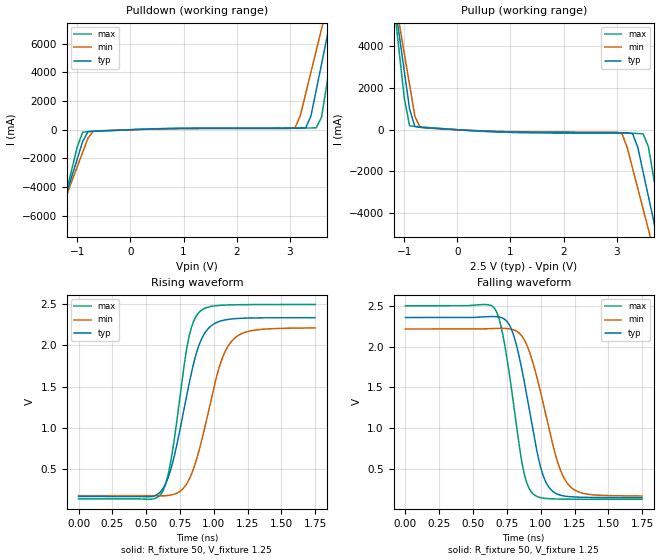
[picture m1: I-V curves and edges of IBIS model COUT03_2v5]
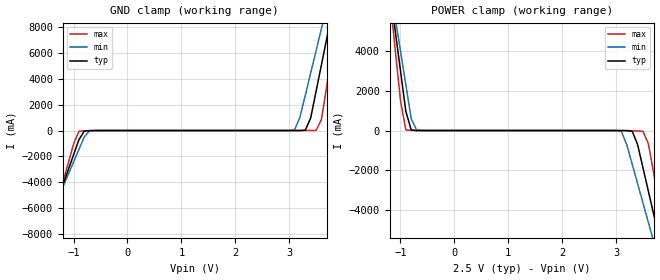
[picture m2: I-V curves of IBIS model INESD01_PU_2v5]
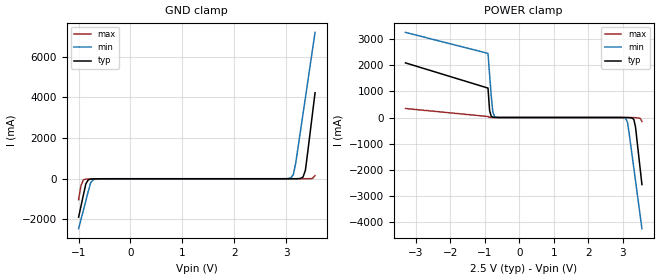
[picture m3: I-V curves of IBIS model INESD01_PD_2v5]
|   This file is an IBIS representation of the   |
|   Integrated Device Technology , Inc.   |
|   ICS8701   |
|   LOW SKEW div1, div2 CLOCK GENERATOR   |
[IBIS Ver]   4.1
[File name]   8701.ibs
[File Rev]   1.0
[Date]   24 Nov 2009 | Last modified
|   Aug 16 2000 | Generated
[Source]   Originated at Integrated Device Technology, Inc.
[Disclaimer]
IDT hereby grants the user of this IBIS model a non-exclusive,
nontransferable license to use this IBIS model under the following terms.
Before using this IBIS model, the user should read this license.
If the user does not accept these terms,  the IBIS model should be
returned to IDT within 30 days.
   The user is granted this license only to use the IBIS model and
is not granted rights to sell, load, rent, lease or license the IBIS
model in whole or in part, or in modified form to anyone other than
user. User may modify the IBIS model to suit its specific
applications but rights to derivative works and such modifications
shall belong to IDT.
   This IBIS model is provided on an "AS IS" basis and IDT makes
absolutely no warranty with respect to the information contained
herein. IDT DISCLAIMS AND CUSTOMER WAIVES ALL WARRANTIES, EXPRESS
OR IMPLIED, INCLUDING WARRANTIES OF MERCHANTABILITY OR FITNESS FOR
A PARTICULAR PURPOSE. The entire risk as to quality and performance
is with the Customer. ACCORDINGLY, IN NO EVENT SHALL THE COMPANY BE
LIABLE FOR ANY DAMAGES, WHETHER IN CONTRACT OR TORT,INCLUDING ANY
LOST PROFITS OR OTHER INCIDENTAL, CONSEQUENTIAL, EXEMPLARY, OR
PUNITIVE DAMAGES ARISING OUT OF THE USE OR APPLICATION OF THE IBIS
model provided in this package. Further, IDT reserves the right to
make changes without notice to any product herein to improve
reliability, function, or design. IDT does not convey any license
under patent rights or any other intellectual property rights,
including those of third parties.
   IDT is not obligated to provide maintenance or support
for the licensed IBIS model.
[Copyright]   Copyright 2002 by Integrated Device Technology , Inc.
[Component]   ICS8701Y
[Manufacturer] Integrated Device Technology, Inc.
[Package]
|LQFP48
|lead + wire   typ   min   max
R_pkg   220.4m   212.5m   238m
L_pkg   1.841nH   1.708nH   1.974n
C_pkg   0.316pF   0.2907pF   0.338pF
[Pin] signal_name   model_name   R_pin   L_pin   C_pin
1   QC3   COUT03   238m   1.974n   0.338p
2   VDDO   POWER   225m   1.831n   0.330p
3   QC4   COUT03   220m   1.781n   0.323p
4   QD0   COUT03   214m   1.732n   0.312p
5   VDDO   POWER   214m   1.709n   0.305p
6   QD1   COUT03   213m   1.708n   0.291p
7   GND   GND   213m   1.708n   0.291p
8   QD2   COUT03   214m   1.709n   0.305p
9   GND   GND   214m   1.732n   0.312p
10   QD3   COUT03   220m   1.781n   0.323p
11   VDDO   POWER   225m   1.831n   0.330p
12   QD4   COUT03   238m   1.974n   0.338p
13   DIV_SELD   INESD01_PU   238m   1.974n   0.338p
14   DIV_SELC   INESD01_PU   225m   1.831n   0.330p
15   nMR/OE   INESD01_PU   220m   1.781n   0.323p
16   VDD   POWER   214m   1.732n   0.312p
17   BANK_EN1   INESD01_PU   214m   1.709n   0.305p
18   GND   GND   213m   1.708n   0.291p
19   BANK_EN0   INESD01_PU   213m   1.708n   0.291p
20   VDD   POWER   214m   1.709n   0.305p
21   GND   GND   214m   1.732n   0.312p
22   CLK   INESD01_PD   220m   1.781n   0.323p
23   DIV_SELB   INESD01_PU   225m   1.831n   0.330p
24   DIV_SELA   INESD01_PU   238m   1.974n   0.338p
25   QA0   COUT03   238m   1.974n   0.338p
26   VDDO   POWER   225m   1.831n   0.330p
27   QA1   COUT03   220m   1.781n   0.323p
28   GND   GND   214m   1.732n   0.312p
29   QA2   COUT03   214m   1.709n   0.305p
30   GND   GND   213m   1.708n   0.291p
31   QA3   COUT03   213m   1.708n   0.291p
32   VDDO   POWER   214m   1.709n   0.305p
33   QA4   COUT03   214m   1.732n   0.312p
34   QB0   COUT03   220m   1.781n   0.323p
35   VDDO   POWER   225m   1.831n   0.330p
36   QB1   COUT03   238m   1.974n   0.338p
37   GND   GND   238m   1.974n   0.338p
38   QB2   COUT03   225m   1.831n   0.330p
39   GND   GND   220m   1.781n   0.323p
40   QB3   COUT03   214m   1.732n   0.312p
41   VDDO   POWER   214m   1.709n   0.305p
42   QB4   COUT03   213m   1.708n   0.291p
43   QC0   COUT03   213m   1.708n   0.291p
44   VDDO   POWER   214m   1.709n   0.305p
45   QC1   COUT03   214m   1.732n   0.312p
46   GND   GND   220m   1.781n   0.323p
47   QC2   COUT03   225m   1.831n   0.330p
48   GND   GND   238m   1.974n   0.338p
[Model Selector] COUT03
COUT03_2v5  Buffer selection for 2v5
COUT03_3v3  Buffer selection for 3v3
[Model Selector] INESD01_PU
INESD01_PU_2v5  Buffer selection for 2v5
INESD01_PU_3v3  Buffer selection for 3v3
[Model Selector] INESD01_PD
INESD01_PD_2v5  Buffer selection for 2v5
INESD01_PD_3v3  Buffer selection for 3v3
| Models and submodels in the file (6): COUT03_2v5 (Output), INESD01_PU_2v5 (Input), INESD01_PD_2v5 (Input), COUT03_3v3 (Output), INESD01_PU_3v3 (Input), INESD01_PD_3v3 (Input)
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[Model] COUT03_2v5
Model_type   Output
Polarity   Non-Inverting
|   typ   min   max
C_comp   2pF   1.5pF   2.5pF
Vmeas = 1.25V
Rref = 50
Cref = 0
Vref = 1.25V
|   typ   min   max
[Voltage range]   2.5V   2.375V   2.625V
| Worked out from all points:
|   slope of the pulldown table from 0 to 0.375 V, typ, clamps not added: 7.86 ohm
|   slope of the pullup table from 0 to 0.375 V, typ, clamps not added: 7.18 ohm
|   rising waveform, R_fixture 50, V_fixture 1.25: 20-80 % time 171ps typ, 188ps min, 123ps max; typ from 0.163 V to 2.34 V
|   falling waveform, R_fixture 50, V_fixture 1.25: 20-80 % time 153ps typ, 185ps min, 125ps max; typ from 2.35 V to 0.154 V
[Pulldown]
|Voltage   I (typ)   I (min)   I (max)
-3.3V     -29.21A    -25.24A    -35.89A
-1.5V     -7.924A    -7.485A    -8.724A
-1.4V     -6.739A    -6.498A    -7.212A
-900mV    -814mA     -1.56A     -170mA
-700mV    -98.53mA   -106.3mA   -114.1mA
3.1V      103.9mA    137.5mA    121.4mA
3.3V      129mA      2.499A     122mA
3.4V      958.9mA    4.006A     122.9mA
3.6V      4.58A      7.024A     878.2mA
3.7V      6.391A     8.534A     3.192A
3.9V      10.02A     11.55A     7.823A
6.6V      59.32A     52.62A     70.8A
[Pullup]
|Voltage   I (typ)   I (min)   I (max)
-3.3V     44.66A     38.54A     54.95A
-1.2V     6.458A     6.703A     6.17A
-1.1V     4.638A     5.186A     3.844A
-1V       2.817A     3.67A      1.518A
-900mV    996.3mA    2.153A     194.9mA
-700mV    116.1mA    120.7mA    136.7mA
3.1V      -144.3mA   -177.7mA   -168.5mA
3.4V      -851mA     -2.819A    -180.7mA
3.6V      -3.21A     -4.786A    -822.6mA
3.7V      -4.391A    -5.77A     -2.33A
3.9V      -6.753A    -7.739A    -5.346A
6.6V      -38.66A    -34.34A    -46.07A
[Ramp]
|   typ   min   max
dV/dt_r   1.743/0.263n   1.634/0.293n   1.896/0.19n
dV/dt_f   1.77/0.231n   1.639/0.28n   1.903/0.187n
R_load =   50.0000
[Rising Waveform]
R_fixture = 50
V_fixture = 1.25   |Vcc_typ
V_fixture_min = 1.1875 |Vcc_min
V_fixture_max = 1.3125 |Vcc_max
C_fixture = 0.0p
| Time   typ   min   max
0s        162.8mV    173.3mV    133.8mV
614.9ps   238.4mV    170.2mV    204.6mV
684.9ps   510.9mV    180.8mV    621.8mV
814.6ps   1.513V     361.6mV    2.092V
853.1ps   1.799V     516.4mV    2.304V
903.9ps   2.06V      804.5mV    2.423V
1.042ns   2.293V     1.748V     2.487V
1.142ns   2.324V     2.07V      2.494V
1.303ns   2.335V     2.187V     2.497V
1.748ns   2.337V     2.213V     2.498V
[Falling Waveform]
R_fixture = 50
V_fixture = 1.25   |Vcc_typ
V_fixture_min = 1.1875 |Vcc_min
V_fixture_max = 1.3125 |Vcc_max
C_fixture = 0.0p
| Time   typ   min   max
0s        2.355V     2.214V     2.498V
662.2ps   2.366V     2.222V     2.456V
721.7ps   2.345V     2.223V     2.13V
798.8ps   2.141V     2.205V     1.303V
874.1ps   1.606V     2.095V     474.6mV
949.5ps   917.4mV    1.762V     192.4mV
1.046ns   319.7mV    1.11V      143.2mV
1.128ns   193.6mV    572.7mV    137.3mV
1.203ns   167.9mV    316.2mV    135.5mV
1.748ns   154.2mV    174.5mV    133.9mV
[Model] INESD01_PU_2v5
Model_type   Input
Polarity   Non-Inverting
Vinl = 1.4V
Vinh = 1.85V
|   typ   min   max
C_comp   2pF   1.5pF   2.5pF
|   typ   min   max
[Voltage range]  2.5V   2.375V   2.625V
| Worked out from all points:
|   GND clamp passes 1 mA (typ) near -0.54 V on its own axis
|   POWER clamp passes 1 mA (typ) near -0.66 V on its own axis
[GND_clamp]
|Voltage   I(typ)   I(min)   I(max)
-2.5V     -19.6A     -17.18A    -23.67A
-1.6V     -8.969A    -8.332A    -10.1A
-1.5V     -7.788A    -7.349A    -8.588A
-900mV    -707.1mA   -1.46A     -57.43mA
-700mV    -7.027mA   -24.05mA   -13.28mA
3.1V      199.2uA    53.94mA    11.78uA
3.3V      28.4mA     2.748A     652.4uA
3.5V      3.045A     6.192A     15.72mA
3.6V      5.115A     7.914A     872.4mA
3.7V      7.185A     9.638A     3.52A
3.9V      11.33A     13.09A     8.818A
5V        34.14A     32.07A     37.99A
[POWER_clamp]
|Voltage   I(typ)   I(min)   I(max)
-1.5V     9.257A     9.207A     9.48A
-1.2V     7.185A     7.484A     6.83A
-1.1V     5.115A     5.761A     4.182A
-900mV    976.9mA    2.318A     34.23mA
-700mV    1.582mA    24.31mA    1.044mA
3.1V      -2.107mA   -51.03mA   -534.5uA
3.3V      -35.62mA   -1.705A    -10.86mA
3.5V      -1.886A    -3.666A    -39.41mA
3.6V      -3.066A    -4.647A    -666.9mA
3.8V      -5.426A    -6.612A    -3.684A
3.9V      -6.607A    -7.595A    -5.193A
5V        -19.6A     -18.41A    -21.79A
[Model] INESD01_PD_2v5
Model_type   Input
Polarity   Non-Inverting
Vinl = 0.8V
Vinh = 2.0V
|   typ   min   max
C_comp   2pF   1.5pF   2.5pF
|   typ   min   max
[Voltage range]  2.5V   2.375V   2.625V
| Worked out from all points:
|   GND clamp passes 1 mA (typ) near -0.55 V on its own axis
|   POWER clamp passes 1 mA (typ) near -0.68 V on its own axis
[GND_clamp]
|Voltage I(typ)   I(min)   I(max)
-1V       -1.886A    -2.451A    -1.028A
-953.5mV  -1.338A    -1.994A    -328mA
-907mV    -789.6mA   -1.537A    -53.04mA
-860.5mV  -251.4mA   -1.081A    -21.51mA
-767.5mV  -17.28mA   -198.8mA   -10.01mA
-674.5mV  -5.28mA    -15.38mA   -3.684mA
3.092V    224.5uA    49.06mA    51.52uA
3.139V    500.8uA    208.3mA    52.98uA
3.185V    1.252mA    774.6mA    56.66uA
3.325V    81.55mA    3.177A     200uA
3.371V    416.9mA    3.978A     464.6uA
3.557V    4.225A     7.185A     159.2mA
[POWER_clamp]
|Voltage   I(typ)   I(min)   I(max)
-3.3V     2.083A     3.246A     343.1mA
-907mV    1.122A     2.445A     37.78mA
-860.5mV  267.5mA    1.644A     5.973mA
-814mV    47.03mA    844mA      1.727mA
-767.5mV  9.66mA     215.3mA    677uA
-674.5mV  960.6uA    12.66mA    131.4uA
3.092V    -1.849mA   -49.09mA   -51.51uA
3.139V    -3.491mA   -186mA     -159.7uA
3.325V    -84.03mA   -1.955A    -5.102mA
3.371V    -365.4mA   -2.411A    -8.31mA
3.51V     -2.01A     -3.782A    -35.44mA
3.557V    -2.558A    -4.239A    -152.3mA
